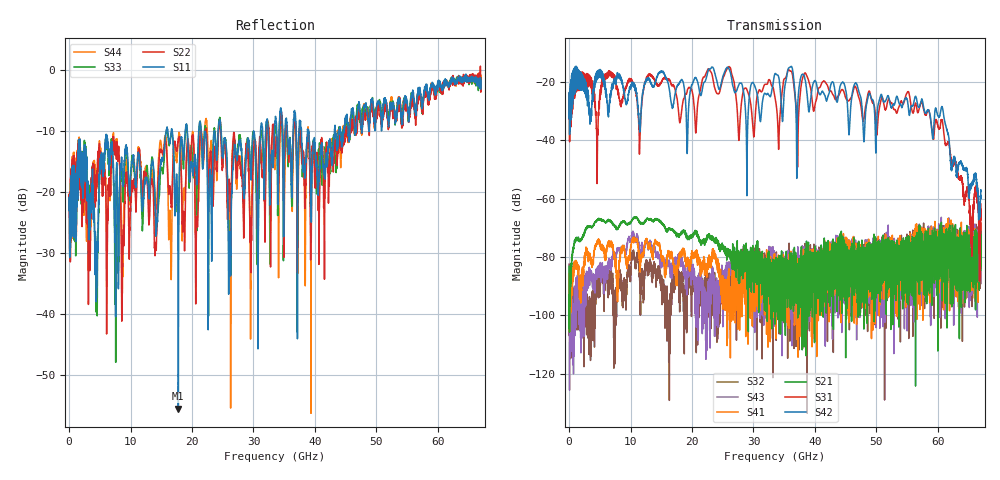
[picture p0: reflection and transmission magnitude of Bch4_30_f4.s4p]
!Agilent Technologies,N5247A,US51170199,A.09.90.13
!Agilent N5247A: A.09.90.13
!Date: Thursday, October 18, 2018 10:20:54
!Correction: S11(Full 4 Port(1,2,3,4))
!S12(Full 4 Port(1,2,3,4))
!S13(Full 4 Port(1,2,3,4))
!S14(Full 4 Port(1,2,3,4))
!S21(Full 4 Port(1,2,3,4))
!S22(Full 4 Port(1,2,3,4))
!S23(Full 4 Port(1,2,3,4))
!S24(Full 4 Port(1,2,3,4))
!S31(Full 4 Port(1,2,3,4))
!S32(Full 4 Port(1,2,3,4))
!S33(Full 4 Port(1,2,3,4))
!S34(Full 4 Port(1,2,3,4))
!S41(Full 4 Port(1,2,3,4))
!S42(Full 4 Port(1,2,3,4))
!S43(Full 4 Port(1,2,3,4))
!S44(Full 4 Port(1,2,3,4))
!S4P File: Measurements: <S11,S12,S13,S14>,
!<S21,S22,S23,S24>,
!<S31,S32,S33,S34>,
!<S41,S42,S43,S44>:
# Hz S  dB  R 50
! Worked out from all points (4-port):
!   6701 points, 10 MHz to 67 GHz, reference 50 ohm
!   strongest paths, dB at 10 MHz, 16.76 GHz, 33.51 GHz, 50.25 GHz, 67 GHz:
!     S42: -32.3, -28.4, -17.1, -28.1, -57.5
!     S31: -32.6, -21.1, -25.3, -33.0, -61.8
!     S21: -83.2, -70.8, -103.0, -92.5, -84.6
!     S41: -85.8, -78.4, -89.9, -80.2, -77.2
!     S43: -88.8, -82.6, -85.4, -80.6, -80.3
!     S32: -82.5, -90.0, -92.1, -77.2, -89.1
!   lowest |S11| = -55.6 dB at 17.78 GHz (marker M1), VSWR 1.00, Z = 50.1 - j0.131 ohm
!   |S11| at or under -10 dB: start of sweep to 15.8 GHz; 24.7 GHz to 31.14 GHz (6.445 GHz wide, 23.1 % of centre); 38.96 GHz to 43.17 GHz (4.206 GHz wide, 10.2 % of centre)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
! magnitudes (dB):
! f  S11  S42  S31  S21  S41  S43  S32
! 10 MHz  -23.0  -32.3  -32.6  -83.2  -85.8  -88.8  -82.5
! 17.78 GHz  -55.6  -20.9  -29.2  -72.3  -81.4  -80.1  -84.0
! 20.77 GHz  -18.8  -19.1  -31.9  -71.0  -78.9  -92.8  -99.9
! 25.98 GHz  -34.9  -15.3  -14.7  -78.5  -87.8  -86.8  -91.1
! 27.65 GHz  -12.3  -20.8  -39.9  -81.4  -92.5  -81.3  -92.0
! 55.1 GHz  -6.1  -26.8  -23.3  -88.2  -84.1  -76.1  -80.2
! 67 GHz  -3.2  -57.5  -61.8  -84.6  -77.2  -80.3  -89.1
